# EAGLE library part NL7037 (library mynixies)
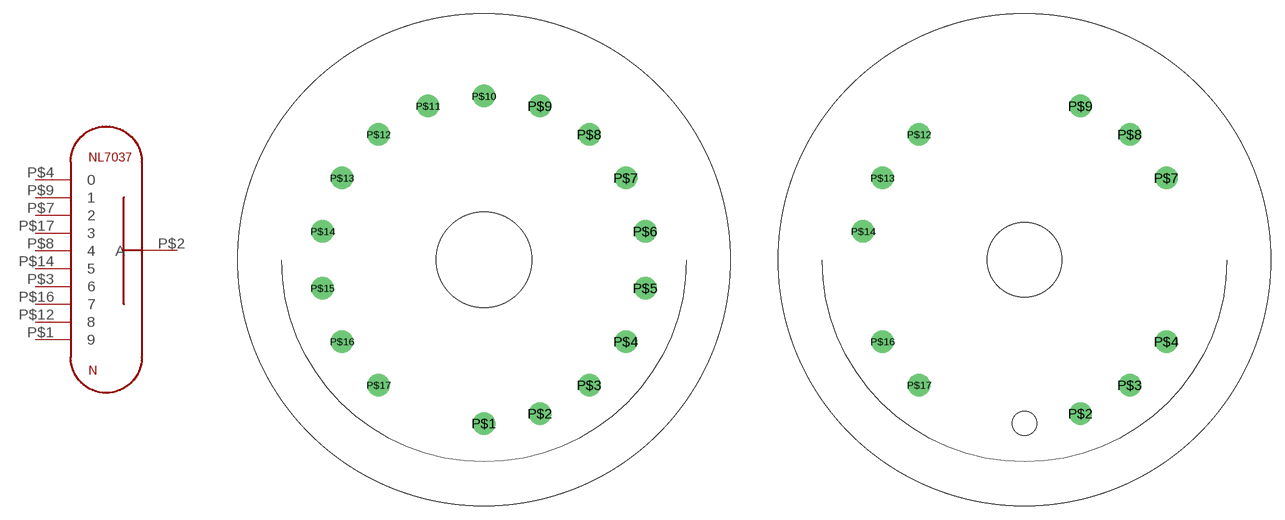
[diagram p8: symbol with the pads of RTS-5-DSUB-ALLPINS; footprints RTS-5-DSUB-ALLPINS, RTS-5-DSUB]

Designator prefix N

## NL7037ALLPINS  [RTS-5-DSUB-ALLPINS]
P$1  9  pas
P$2  A  pas
P$3  6  pas
P$4  0  pas
P$7  2  pas
P$8  4  pas
P$9  1  pas
P$12  8  pas
P$14  5  pas
P$16  7  pas
P$17  3  pas

## NL7037  [RTS-5-DSUB]
P$2  A  pas
P$3  6  pas
P$4  0  pas
P$7  2  pas
P$8  4  pas
P$9  1  pas
P$12  8  pas
P$13  9  pas
P$14  5  pas
P$16  7  pas
P$17  3  pas

## Footprint RTS-5-DSUB-ALLPINS (pad centres in mm)
drill 1.6: P$1 0,-17.462; P$2 5.973,-16.409; P$3 11.225,-13.377; P$4 15.123,-8.731; P$5 17.197,-3.032; P$6 17.197,3.032; P$7 15.123,8.731; P$8 11.225,13.377; P$9 5.973,16.409; P$10 0,17.462; P$11 -5.973,16.409; P$12 -11.225,13.377; P$13 -15.123,8.731; P$14 -17.197,3.032; P$15 -17.197,-3.032; P$16 -15.123,-8.731; P$17 -11.225,-13.377
hole 10.16 at 0,0

## Footprint RTS-5-DSUB (pad centres in mm)
drill 1.6: P$2 5.973,-16.409; P$3 11.225,-13.377; P$4 15.123,-8.731; P$7 15.123,8.731; P$8 11.225,13.377; P$9 5.973,16.409; P$12 -11.225,13.377; P$13 -15.123,8.731; P$14 -17.197,3.032; P$16 -15.123,-8.731; P$17 -11.225,-13.377
hole 7.938 at 0,0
